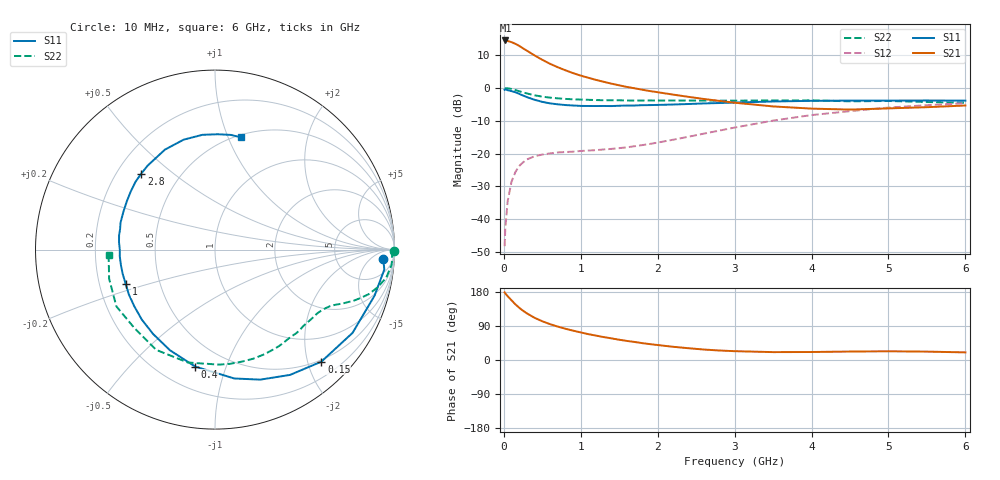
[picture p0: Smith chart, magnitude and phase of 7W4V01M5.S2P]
! Infineon Technologies  Discrete & RF Semiconductors
! BFS17W
! Si NPN RF Bipolar Junction Transistor in SOT323
! VCE = 4 V  IC = 1.5 mA
! Common Emitter S-Parameters:  August  1999
# GHz  S  MA  R  50
!  f  S11  S21  S12  S22
! GHz  MAG  ANG  MAG  ANG  MAG  ANG  MAG  ANG
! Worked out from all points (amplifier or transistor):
!   36 points, 10 MHz to 6 GHz, reference 50 ohm
!   highest |S21| = 14.5 dB at 20 MHz (marker M1)
!   |S21| within 3 dB of that: start of sweep to 291.6 MHz
!   unconditionally stable (mu >= 1): 916.1 MHz to end of sweep
!   at 250 MHz: K = 0.31, MSG = 17.4 dB, |S12| = -22.6 dB
!   at 1.4 GHz: K = 1.29, MAG = 6.7 dB, |S12| = -18.6 dB
!   at 6 GHz: K = 1.09, MAG = -2.2 dB, |S12| = -4.6 dB
!   S11 on the Smith chart (normalised r, x): 10 MHz: 18, -16; 150 MHz: 0.47, -2.25; 400 MHz: 0.34, -0.79; 1 GHz: 0.31, -0.17; 2.8 GHz: 0.30, +0.39; 6 GHz: 0.53, +1.12
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0.01  0.9388 -3.2  5.261 178.4  0.0039 84.4  0.9996 -0.5
0.02  0.9499 -6.7  5.294 175.4  0.0076 87.8  0.9875 -1.8
0.05  0.9253 -16.1  5.198 168.3  0.019 80.2  0.9882 -4.8
0.1  0.8958 -31.2  4.987 157.5  0.0375 72.7  0.967 -9.3
0.15  0.8608 -46.5  4.708 146.9  0.0524 64.6  0.9295 -13.1
0.2  0.8137 -59.1  4.377 137.9  0.0649 59.3  0.8929 -16.1
0.25  0.7671 -70.8  4.015 130.0  0.0738 53.3  0.8561 -18.3
0.3  0.726 -81.5  3.696 123.0  0.0816 49.2  0.8257 -20.1
0.4  0.661 -99.6  3.13 111.3  0.0914 43.3  0.7736 -22.8
0.5  0.6144 -114.1  2.686 102.2  0.0969 39.7  0.7381 -24.6
0.6  0.5832 -126.2  2.336 94.6  0.101 37.5  0.7125 -26.3
0.7  0.5644 -136.2  2.073 88.2  0.1043 37.0  0.6958 -28.1
0.8  0.5496 -144.9  1.861 82.5  0.1058 36.5  0.682 -30.0
1  0.5333 -158.7  1.543 72.8  0.1098 38.3  0.6668 -33.8
1.1  0.5318 -165.2  1.428 68.1  0.1115 39.3  0.6604 -36.2
1.6  0.5406 171.3  1.037 50.3  0.1248 49.1  0.6452 -48.3
2.2  0.5601 151.3  0.793 34.9  0.163 60.5  0.6448 -64.7
2.8  0.5901 134.1  0.636 25.1  0.2242 64.7  0.6419 -82.5
3.5  0.623 116.6  0.524 20.8  0.3185 62.3  0.647 -103.5
4.5  0.6433 96.2  0.469 22.3  0.4437 50.3  0.6266 -135.9
5.5  0.6451 82.1  0.51 22.1  0.5472 37.2  0.6118 -164.6
6  0.6416 76.8  0.541 20.1  0.5874 30.9  0.5935 -177.2
